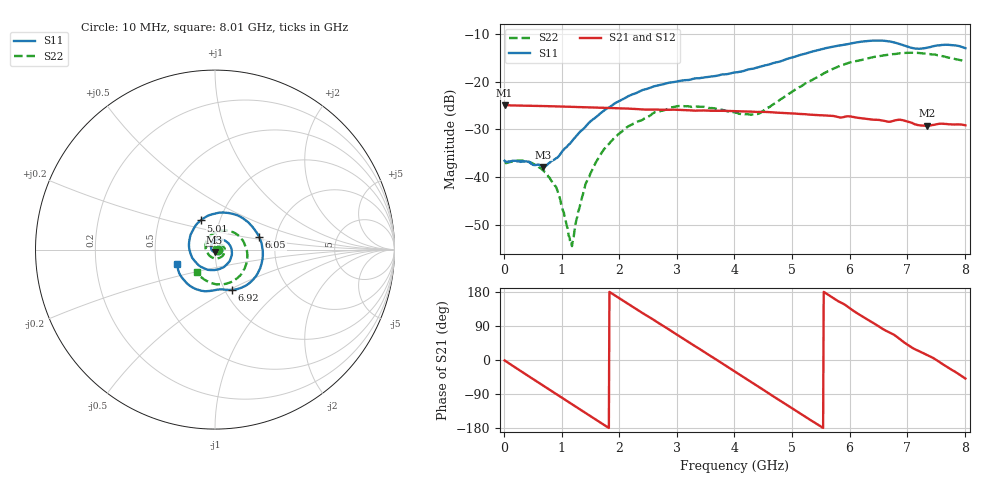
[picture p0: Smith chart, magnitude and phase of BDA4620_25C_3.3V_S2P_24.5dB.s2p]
!Agilent Technologies,E5071B,MY42404982,A.09.10
!Date: Wed May 06 08:54:08 2026
!Data & Calibration Information:
!Freq	S11:SOLT2(ON)	S21:SOLT2(ON)	S12:SOLT2(ON)	S22:SOLT2(ON)
# Hz S RI R 50
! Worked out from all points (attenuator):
!   801 points, 10 MHz to 8.01 GHz, reference 50 ohm
!   highest |S21| = -24.88 dB at 10 MHz (marker M1); lowest = -29.2 dB at 7.34 GHz (marker M2)
!   lowest |S11| = -37.9 dB at 680 MHz (marker M3), VSWR 1.03, Z = 49.7 - j1.24 ohm
!   |S11| at or under -10 dB: start of sweep to end of sweep
!   |S22| runs from -54.5 to -13.9 dB; largest |S21 - S12| = 0.00027
!   S11 on the Smith chart (normalised r, x): 10 MHz: 1.03, -0.00; 5.01 GHz: 0.81, +0.27; 6.05 GHz: 1.63, +0.25; 6.92 GHz: 1.08, -0.52; 8.01 GHz: 0.64, -0.11
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1e7  0.0148 -0.000949  0.057 -0.00121  0.057 -0.00121  0.014 -0.000401
4.1e8  0.00866 -0.0116  0.0424 -0.0369  0.0424 -0.037  0.0137 -0.0049
6.8e8  -0.00272 -0.0125  0.0212 -0.0515  0.0211 -0.0516  0.00939 -0.00698
9.2e8  -0.0145 -0.00646  -0.00134 -0.0552  -0.00143 -0.0553  0.00371 -0.00637
1.16e9  -0.0217 0.00795  -0.0231 -0.0496  -0.0232 -0.0496  -0.00158 -0.00118
1.2e9  -0.0222 0.0109  -0.0264 -0.0478  -0.0265 -0.0479  -0.00221 -2.99e-05
1.35e9  -0.0217 0.0222  -0.0375 -0.0393  -0.0375 -0.0393  -0.00372 0.00464
1.53e9  -0.0154 0.0366  -0.0472 -0.026  -0.0472 -0.026  -0.0035 0.0113
1.77e9  0.00222 0.0515  -0.053 -0.0051  -0.0531 -0.00507  0.000654 0.0206
2.15e9  0.0447 0.0543  -0.0447 0.0274  -0.0447 0.0274  0.017 0.0293
2.68e9  0.0922 0.0026  -0.007 0.0506  -0.00698 0.0507  0.0444 0.0196
3.08e9  0.0822 -0.0626  0.0259 0.0436  0.0261 0.0436  0.0554 -0.00739
4.01e9  -0.0892 -0.0884  0.0424 -0.0253  0.0425 -0.0253  -0.0105 -0.0468
4.42e9  -0.1433 0.00362  0.0161 -0.0456  0.0161 -0.0456  -0.0447 -0.0128
5.01e9  -0.0799 0.1624  -0.0288 -0.0365  -0.0289 -0.0366  -0.0303 0.0736
5.35e9  0.0287 0.2061  -0.0427 -0.0146  -0.0428 -0.0146  0.0228 0.1021
6.05e9  0.2454 0.0714  -0.0284 0.0322  -0.0284 0.0322  0.1538 0.0525
6.68e9  0.1877 -0.1898  0.0108 0.0365  0.0108 0.0366  0.1704 -0.0905
6.92e9  0.0959 -0.225  0.0258 0.0301  0.0258 0.0301  0.1413 -0.1434
7.34e9  -0.0122 -0.2278  0.0336 0.0081  0.0337 0.00815  0.0426 -0.1934
7.66e9  -0.1295 -0.2088  0.0348 -0.00959  0.0348 -0.00957  -0.0354 -0.1804
8.01e9  -0.2107 -0.0819  0.0229 -0.0264  0.023 -0.0264  -0.1022 -0.1275
